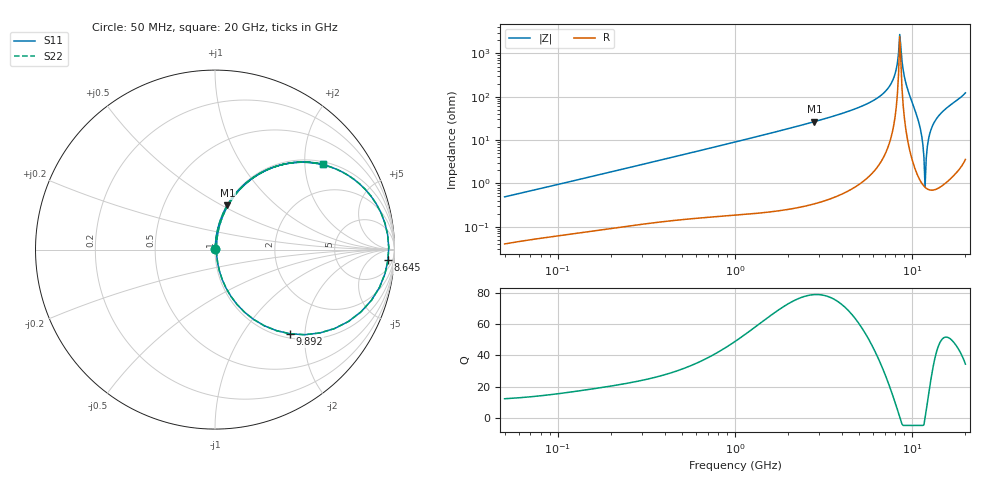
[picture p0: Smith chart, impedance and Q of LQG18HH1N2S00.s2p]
!Murata Part Number: LQG18HH1N2S00
!These Parameters are Measured in Series Mode Connection
!  o--[Z]--o
!Port1  Port2
!  o-------o
!Freq. Start=50[MHz] Stop=20[GHz], 401[Steps]
# Hz S RI R 50
!Freq.(Hz) S11(Real) S11(Imag) S21(Real) S21(Imag) S12(Real) S12(Imag) S22(Real) S22(Imag)
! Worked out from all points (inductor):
!   401 points, 50 MHz to 20 GHz, reference 50 ohm
!   read as one part in series: L = 1.53 nH near 51.52 MHz
!   highest Q = 79.1 at 2.811 GHz (marker M1), where L = 1.51 nH
!   self-resonance near 8.516 GHz
!   S11 on the Smith chart (normalised r, x): 50 MHz: 1.00, +0.01; 8.645 GHz: 14, -25; 9.892 GHz: 1.08, -1.68; 20 GHz: 1.07, +2.46
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5e7  0.000423 0.00486  0.9996 -0.00486  0.9996 -0.00486  0.000423 0.00486
1.364002e8  0.000889 0.0127  0.9991 -0.0127  0.9991 -0.0127  0.000889 0.0127
3.721004e8  0.00241 0.0337  0.9976 -0.0337  0.9976 -0.0337  0.00241 0.0337
1e9  0.00985 0.0891  0.9901 -0.0891  0.9901 -0.0891  0.00985 0.0891
2.728004e9  0.065 0.2403  0.935 -0.2403  0.935 -0.2403  0.065 0.2403
2.810964e9  0.0691 0.2474  0.9309 -0.2474  0.9309 -0.2474  0.0691 0.2474
5.194772e9  0.2715 0.4362  0.7285 -0.4362  0.7285 -0.4362  0.2715 0.4362
7.442007e9  0.7403 0.4147  0.2597 -0.4147  0.2597 -0.4147  0.7403 0.4147
8.020766e9  0.899 0.2542  0.101 -0.2542  0.101 -0.2542  0.899 0.2542
8.389408e9  0.9617 0.084  0.0383 -0.084  0.0383 -0.084  0.9617 0.084
8.644534e9  0.9636 -0.059  0.0364 0.059  0.0364 0.059  0.9636 -0.059
9.178299e9  0.8136 -0.3468  0.1864 0.3468  0.1864 0.3468  0.8136 -0.3468
9.892087e9  0.4189 -0.4692  0.5811 0.4692  0.5811 0.4692  0.4189 -0.4692
1.098561e10  0.0607 -0.2128  0.9393 0.2128  0.9393 0.2128  0.0607 -0.2128
1.131968e10  0.0256 -0.1229  0.9744 0.1229  0.9744 0.1229  0.0256 -0.1229
1.149051e10  0.0158 -0.0802  0.9842 0.0802  0.9842 0.0802  0.0158 -0.0802
1.183995e10  0.00807 -0.000598  0.9919 0.000598  0.9919 0.000598  0.00807 -0.000598
1.220001e10  0.0124 0.0707  0.9876 -0.0707  0.9876 -0.0707  0.0124 0.0707
1.238412e10  0.018 0.1033  0.982 -0.1033  0.982 -0.1033  0.018 0.1033
1.276073e10  0.0343 0.1627  0.9657 -0.1627  0.9657 -0.1627  0.0343 0.1627
1.375312e10  0.0952 0.282  0.9048 -0.282  0.9048 -0.282  0.0952 0.282
2e10  0.5995 0.4757  0.4005 -0.4757  0.4005 -0.4757  0.5995 0.4757
